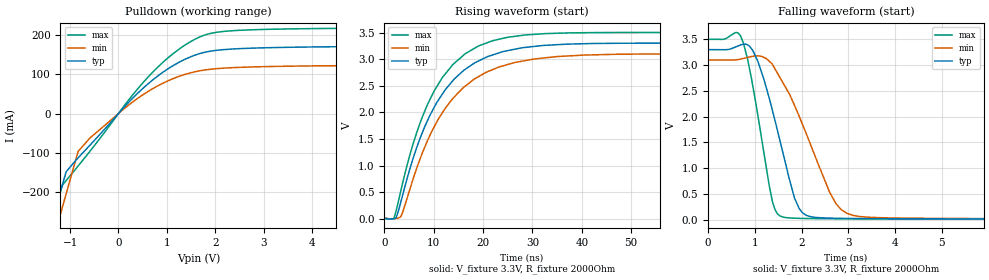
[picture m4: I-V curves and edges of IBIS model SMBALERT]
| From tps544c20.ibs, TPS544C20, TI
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|   Model
[Model]   SMBALERT
Model_type   Open_drain
Polarity   Non-Inverting
Vmeas = 1.65
Vref = 3.3
Cref = 1pF
Rref = 2000
|   typ   min   max
C_comp   2.817pF   2.476pF   3.036pF
[Voltage Range]   3.3   3.1   3.5
[Temperature Range]   25   125   -40
[Pullup Reference]   3.3   3.1   3.5
[Pulldown Reference]   0   0   0
[Power Clamp Reference]   3.3   3.1   3.5
[GND Clamp Reference]   0   0   0
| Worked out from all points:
|   slope of the pulldown table from 0 to 0.495 V, typ, clamps not added: 7.88 ohm
|   falling waveform, V_fixture 3.3V, R_fixture 2000Ohm: 20-80 % time 554ps typ, 844ps min, 386ps max; typ from 3.3 V to 0.012 V
|   rising waveform, V_fixture 3.3V, R_fixture 2000Ohm: 20-80 % time 9.98ns typ, 10.8ns min, 9.23ns max; typ from 0.012 V to 3.3 V
[Pulldown]
|   Voltage   I(typ)   I(min)   I(max)
-3.3V     -1.189A    -1.25A     -1.154A
-1.825V   -467.2mA   -529mA     -430.9mA
-1.161V   -181.9mA   -238.7mA   -182.5mA
-1.082V   -148.3mA   -204.6mA   -170.8mA
-834.9mV  -112.7mA   -96.47mA   -133.7mA
-587.4mV  -80.3mA    -62.04mA   -95.75mA
224.4mV   30.26mA    22.8mA     36.67mA
699.6mV   84.55mA    62.6mA     104.1mA
1.254V    130.5mA    94.56mA    163.9mA
1.719V    153.9mA    109.5mA    196.8mA
2.779V    166.4mA    118.5mA    213.1mA
6.6V      171.9mA    123.5mA    218.7mA
[Ramp]
R_load = 2000
|   typ   min   max
dV/dt_r   1.97304/9.98445e-09   1.85122/1.08064e-08   2.09392/9.23026e-09
dV/dt_f   1.973/5.53534e-10   1.85118/8.39315e-10   2.09389/3.85769e-10
[Falling Waveform]
V_fixture = 3.3V
V_fixture_min = 3.1V
V_fixture_max = 3.5V
R_fixture = 2000Ohm
C_fixture = 0F
|   Time   V(typ)   V(min)   V(max)
0s        3.3V       3.1V       3.5V
645.6ps   3.373V     3.108V     3.622V
757.3ps   3.407V     3.13V      3.424V
954.6ps   3.287V     3.17V      2.607V
1.378ns   2.113V     3.009V     342.5mV
1.833ns   471.9mV    2.25V      27.21mV
2.104ns   81.09mV    1.658V     20.92mV
2.738ns   25.44mV    306.8mV    15.47mV
3.612ns   17.81mV    38.45mV    12.5mV
100ns     11.66mV    14.42mV    10.28mV
[Rising Waveform]
V_fixture = 3.3V
V_fixture_min = 3.1V
V_fixture_max = 3.5V
R_fixture = 2000Ohm
C_fixture = 0F
|   Time   V(typ)   V(min)   V(max)
0s        11.66mV    14.42mV    10.28mV
1.953ns   5.067mV    8.331mV    18.34mV
3.413ns   341.4mV    56.58mV    554.7mV
6.592ns   1.348V     960.6mV    1.63V
10.09ns   2.093V     1.728V     2.402V
13.86ns   2.594V     2.262V     2.897V
19.06ns   2.965V     2.672V     3.248V
26.33ns   3.186V     2.936V     3.428V
35.02ns   3.273V     3.05V      3.487V
100ns     3.3V       3.1V       3.5V
